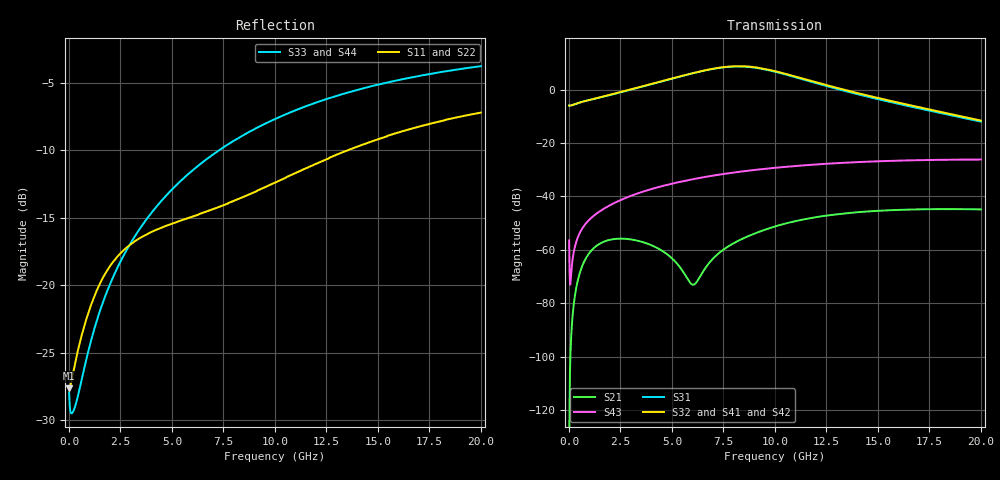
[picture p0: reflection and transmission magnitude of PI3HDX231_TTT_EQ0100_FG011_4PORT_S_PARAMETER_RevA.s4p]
! NPort=4 DATA=2000 NOISE=0 GROUPDELAY=0 COMPLEX_DATAFORMAT=POLAR
! NumOfBlock=1 NumOfParam=0
! .MODEL Smodel S TSTONEFILE=PI3HDX231_TTT_EQ0100_FG011_4PORT_S_PARAMETER_RevA.s4p TYPE=S
!  -- The above .MODEL line can be used for the S element in the netlist.
! The s parameter is extracted from the linear redriver, it is not bi-directional; only s(4,1)s(4,2) and s(3,1)s(3,2)
! should be the insertion loss
!Port definition:
!Port1 = input+
!Port2 = input-
!Port3 = output+
!Port4 = output-
# Hz S MA R  50
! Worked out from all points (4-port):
!   2000 points, 10 MHz to 20 GHz, reference 50 ohm
!   strongest paths, dB at 10 MHz, 5.01 GHz, 10.01 GHz, 15.01 GHz, 20 GHz:
!     S32: -5.9, 4.2, 6.9, -3.2, -11.6
!     S41: -5.9, 4.2, 6.9, -3.3, -11.7
!     S42: -5.9, 4.2, 6.8, -3.4, -11.6
!     S31: -5.9, 4.1, 6.7, -3.6, -12.0
!     S43: -56.5, -35.2, -29.3, -26.9, -26.2
!     S21: -134.8, -63.2, -51.3, -45.4, -44.9
!   lowest |S11| = -27.6 dB at 10 MHz (marker M1), VSWR 1.09, Z = 46 - j0.0776 ohm
!   |S11| at or under -10 dB: start of sweep to 13.55 GHz
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1e7  0.04152 -178.8  1.825e-07 -13.9  0 0.0  0 0.0
     1.825e-07 -14.0  0.04152 -178.8  0 0.0  0 0.0
     0.5042 -0.5  0.5042 179.5  0.04012 -3.2  0.0015 -70.3
     0.5042 179.5  0.5042 -0.5  0.0015 -70.3  0.04012 -3.2
5.28e9  0.172 -139.6  0.0005308 -12.7  7.924e-10 -177.5  3.913e-10 -153.0
        0.0005338 -12.4  0.172 -139.7  3.774e-10 -152.6  8.264e-10 -177.7
        1.716 -56.3  1.722 123.2  0.2375 -103.3  0.01835 60.0
        1.725 122.9  1.738 -55.3  0.0183 60.0  0.2375 -103.3
7.28e9  0.1948 -135.2  0.0008683 101.3  5.99e-09 118.7  2.549e-09 178.2
        0.0008648 100.4  0.1944 -135.4  2.477e-09 179.7  6.267e-09 117.4
        2.541 -113.4  2.561 66.2  0.3154 -108.8  0.02556 48.1
        2.561 65.8  2.582 -112.4  0.02547 48.1  0.3155 -108.8
8.88e9  0.219 -131.5  0.001934 92.7  1.781e-08 65.5  1.116e-08 137.3
        0.00192 92.2  0.2181 -131.8  1.096e-08 139.0  1.851e-08 63.3
        2.616 -171.7  2.658 7.8  0.3737 -112.9  0.03094 37.8
        2.653 7.5  2.661 -170.6  0.03082 37.9  0.3739 -112.9
1.057e10  0.2513 -128.9  0.003166 77.5  3.834e-08 19.3  3.15e-08 80.7
          0.003143 77.1  0.2499 -129.1  3.115e-08 82.5  3.919e-08 16.5
          1.893 133.3  1.945 -47.4  0.4304 -117.0  0.036 26.8
          1.937 -47.8  1.927 134.6  0.03587 26.9  0.4305 -117.0
1.32e10  0.3087 -128.2  0.00475 50.4  9.67e-08 -38.0  8.193e-08 5.7
         0.004711 50.1  0.3068 -128.2  8.179e-08 7.4  9.706e-08 -40.7
         0.9856 73.7  1.03 -108.2  0.5075 -122.9  0.04236 9.6
         1.021 -108.6  1.008 75.2  0.04227 9.8  0.5074 -122.9
2e10  0.4355 -135.6  0.005752 -4.6  3.792e-07 -160.2  2.789e-07 -133.4
      0.005704 -4.8  0.4338 -135.4  2.812e-07 -132.4  3.726e-07 -162.3
      0.2513 -34.0  0.2628 139.6  0.6464 -135.0  0.04883 -32.3
      0.2592 139.7  0.2617 -32.4  0.04894 -32.0  0.6461 -135.0
